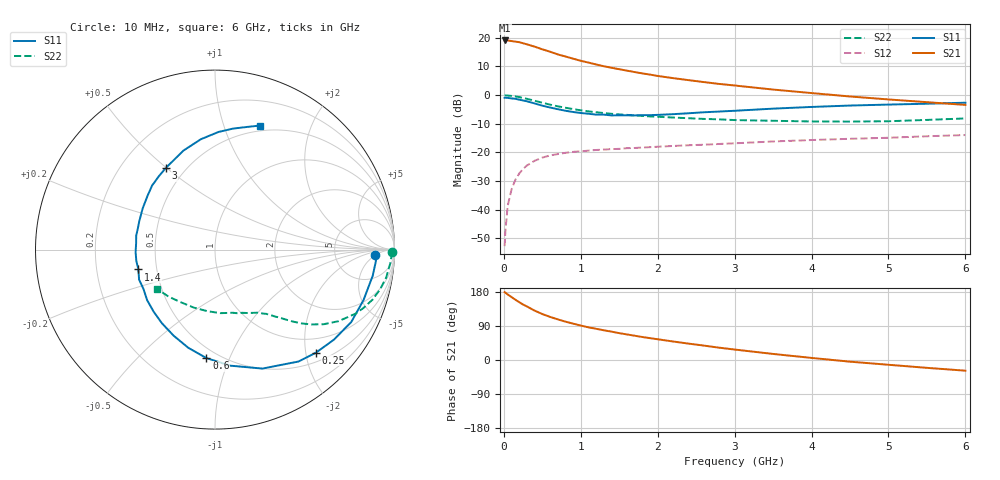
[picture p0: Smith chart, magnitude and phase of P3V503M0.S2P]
! SIEMENS Small Signal Semiconductors
! BFP181
! Si NPN RF Bipolar Junction Transistor in SOT143
! VCE = 0.5 V  IC = 3 mA
! Common Emitter S-Parameters:  March  1996
# GHz  S  MA  R  50
!  f  S11  S21  S12  S22
! GHz  MAG  ANG  MAG  ANG  MAG  ANG  MAG  ANG
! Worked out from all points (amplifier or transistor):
!   36 points, 10 MHz to 6 GHz, reference 50 ohm
!   highest |S21| = 19.1 dB at 10 MHz (marker M1)
!   |S21| within 3 dB of that: start of sweep to 490.1 MHz
!   unconditionally stable (mu >= 1): 1.55 GHz to end of sweep
!   at 250 MHz: K = 0.20, MSG = 21.9 dB, |S12| = -25.8 dB
!   at 1.4 GHz: K = 0.94, MSG = 14.2 dB, |S12| = -18.9 dB
!   at 6 GHz: K = 1.33, MAG = 1.8 dB, |S12| = -14.0 dB
!   S11 on the Smith chart (normalised r, x): 10 MHz: 16, -5; 250 MHz: 0.68, -2.20; 600 MHz: 0.43, -0.83; 1.4 GHz: 0.39, -0.11; 3 GHz: 0.39, +0.50; 6 GHz: 0.44, +1.33
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0.01  0.8937 -2.1  8.974 178.9  0.0023 84.7  0.984 -0.8
0.02  0.8991 -3.9  8.94 177.7  0.0042 86.2  0.9853 -1.9
0.05  0.8908 -9.4  8.951 173.0  0.0116 85.8  0.9788 -4.7
0.1  0.874 -18.8  8.762 166.0  0.0225 77.9  0.9665 -9.3
0.15  0.8597 -28.0  8.561 159.1  0.0332 73.0  0.9463 -13.5
0.2  0.8312 -37.1  8.372 152.6  0.0427 68.8  0.9211 -17.6
0.25  0.8038 -45.6  8.009 146.3  0.0513 64.1  0.8895 -21.4
0.4  0.7135 -68.3  6.999 130.3  0.0712 52.8  0.7954 -30.1
0.5  0.6522 -82.5  6.286 121.3  0.0808 47.0  0.7342 -34.5
0.6  0.6063 -94.5  5.712 113.8  0.0882 42.4  0.6802 -37.8
0.7  0.567 -105.2  5.129 107.3  0.0931 38.9  0.6363 -40.3
0.8  0.5324 -115.6  4.713 101.3  0.098 36.1  0.6006 -42.2
1  0.4862 -134.7  3.962 90.9  0.1041 31.6  0.5412 -45.4
1.1  0.4714 -143.4  3.688 86.2  0.1071 30.0  0.5189 -46.7
1.4  0.441 -165.5  2.996 74.8  0.1138 26.3  0.471 -50.4
1.8  0.4459 169.9  2.387 60.7  0.1212 24.0  0.4321 -54.8
2.2  0.4636 150.4  1.974 48.8  0.1291 21.6  0.4052 -60.5
3  0.5315 120.9  1.468 27.6  0.1437 18.1  0.3658 -74.2
3.5  0.5789 107.7  1.247 16.0  0.1547 16.0  0.3554 -85.0
4.5  0.6557 88.3  0.944 -4.4  0.1723 10.1  0.3441 -110.0
5.5  0.7056 75.5  0.751 -20.7  0.1907 5.6  0.368 -134.5
6  0.7349 70.1  0.673 -28.2  0.2004 2.5  0.3908 -146.1
